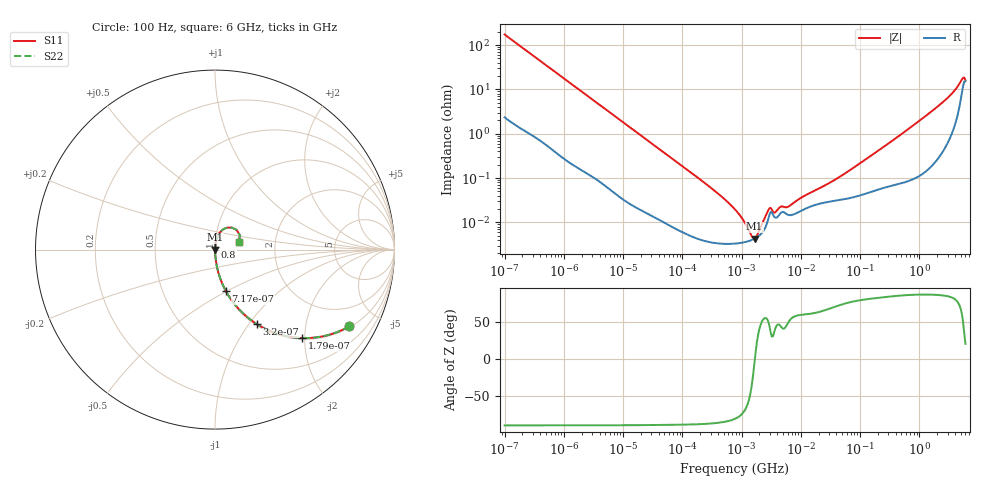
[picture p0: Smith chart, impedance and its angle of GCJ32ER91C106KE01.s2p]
!Murata Part Number: GCJ32ER91C106KE01
!These Parameters are Measured in Series Mode Connection
!Data Generated on Mar 13, 2026
!  o--ll--o
!Port1  Port2
!  o------o
!Operation Temp=25[degC], DC Bias Voltage=0[V]
!Freq. Start=100[Hz] Stop=6[GHz] 401[Steps]
# Hz S RI R 50
!Freq.(Hz) S11(Real) S11(Imag) S21(Real) S21(Imag) S12(Real) S12(Imag) S22(Real) S22(Imag)
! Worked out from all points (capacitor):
!   401 points, 100 Hz to 6 GHz, reference 50 ohm
!   read as one part in series: C = 9.14 uF near 109 Hz
!   lowest |Z| = 4.31 mohm at 1.658 MHz (marker M1)
!   series resonance near 1.676 MHz, so ESL is about 990 pH
!   S11 on the Smith chart (normalised r, x): 100 Hz: 1.05, -3.47; 179 Hz: 1.03, -1.95; 320 Hz: 1.02, -1.10; 717 Hz: 1.01, -0.49; 800 MHz: 1.00, +0.03; 6 GHz: 1.30, +0.11
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100  0.7481 -0.4274  0.2519 0.4274  0.2519 0.4274  0.7481 -0.4274
179  0.4874 -0.4929  0.5126 0.4929  0.5126 0.4929  0.4874 -0.4929
320  0.2342 -0.4158  0.7658 0.4158  0.7658 0.4158  0.2342 -0.4158
717  0.0606 -0.2309  0.9394 0.2309  0.9394 0.2309  0.0606 -0.2309
2008  0.0093 -0.088  0.9907 0.088  0.9907 0.088  0.0093 -0.088
40335  0.000136 -0.00458  0.9999 0.00458  0.9999 0.00458  0.000136 -0.00458
316350  3.54e-05 -0.000577  1 0.000577  1 0.000577  3.54e-05 -0.000577
774597  3.33e-05 -0.000194  1 0.000194  1 0.000194  3.33e-05 -0.000194
1159002  3.61e-05 -8.7e-05  1 8.7e-05  1 8.7e-05  3.61e-05 -8.7e-05
1658239  4.3e-05 -2.5e-06  1 2.5e-06  1 2.5e-06  4.3e-05 -2.5e-06
2169299  5.66e-05 6.56e-05  0.9999 -6.56e-05  0.9999 -6.56e-05  5.66e-05 6.56e-05
2967816  0.000151 0.000145  0.9998 -0.000145  0.9998 -0.000145  0.000151 0.000145
3712478  0.000128 0.000112  0.9999 -0.000112  0.9999 -0.000112  0.000128 0.000112
4643984  0.000166 0.000157  0.9998 -0.000157  0.9998 -0.000157  0.000166 0.000157
6075234  0.000148 0.000169  0.9999 -0.000169  0.9999 -0.000169  0.000148 0.000169
1.555665e7  0.000235 0.00043  0.9998 -0.00043  0.9998 -0.00043  0.000235 0.00043
4.764863e7  0.000325 0.00106  0.9997 -0.00106  0.9997 -0.00106  0.000325 0.00106
3.124326e8  0.000689 0.0062  0.9993 -0.0062  0.9993 -0.0062  0.000689 0.0062
8.000355e8  0.0012 0.0156  0.9988 -0.0156  0.9988 -0.0156  0.0012 0.0156
3.666503e9  0.0179 0.0813  0.9821 -0.0813  0.9821 -0.0813  0.0179 0.0813
5.245841e9  0.0943 0.1224  0.9057 -0.1224  0.9057 -0.1224  0.0943 0.1224
6e9  0.1342 0.0427  0.8658 -0.0427  0.8658 -0.0427  0.1342 0.0427
